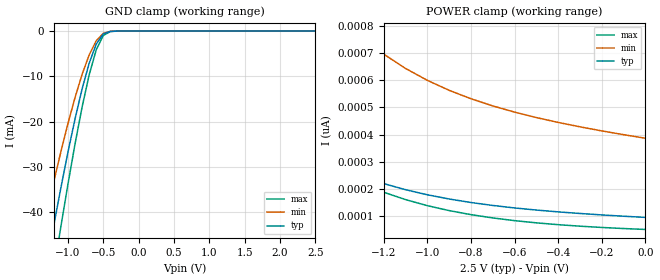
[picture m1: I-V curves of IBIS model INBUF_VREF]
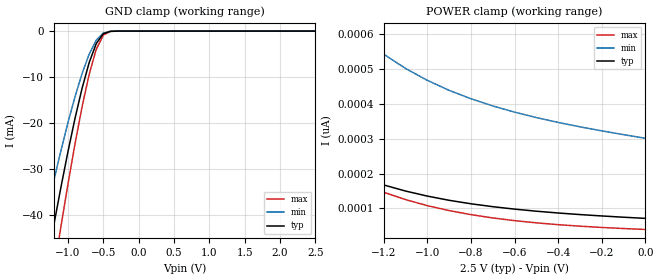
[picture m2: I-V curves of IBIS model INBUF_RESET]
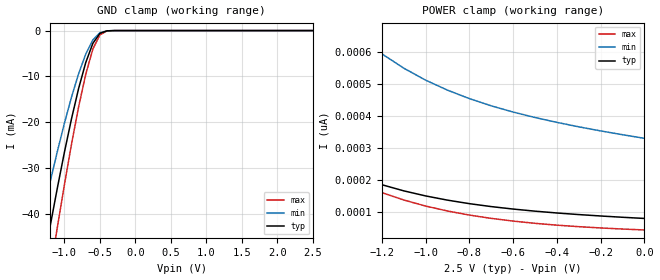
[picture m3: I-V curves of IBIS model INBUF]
| IBIS file sstvn859_mlf_2700.ibs created by s2ibis2 version 1.2
| North Carolina State University Electronics Research Laboratory  1995
[IBIS ver]   2.1
[File name]   sstvn859_mlf_2700.ibs
[File Rev]   1.0
[Date]   Thursday, November 6, 2003
[Source]   IDT
[Notes]   1. Temp typ=25C, min=0C, max=70C
   2. IDT's 2.0v C11.5 process
   3. Ramp rate based on 50 ohm load
READ THESE TERMS AND CONDITIONS CAREFULLY BEFORE USING THIS IBIS MODEL.  BY
USING THIS IBIS MODEL, YOU ARE ACCEPTING AND AGREEING TO THESE TERMS AND
CONDITIONS OF USE.
Integrated Device Technology, Inc. ("IDT") hereby grants the user of this
IBIS model ("User") a non-exclusive, nontransferable license to use this
IBIS model under the following terms: The User is granted this license only
to use the IBIS model for demonstration purposes only and is not granted
rights to sell, copy (except as needed to run the IBIS model), rent, lease
or sub-license (except for demonstration) the IBIS model in whole or in
part, or in modified form to anyone. The User may modify the IBIS model to
suit its specific applications, but  rights to derivative works and such
modifications shall belong to IDT.
THIS IBIS MODEL IS PROVIDED ON AN AS IS" BASIS AND IDT  MAKES ABSOLUTELY NO
WARRANTY WITH RESPECT TO THE INFORMATION CONTAINED HEREIN.  IDT DISCLAIMS
AND USER WAIVES ALL WARRANTIES, EXPRESS AND IMPLIED, INCLUDING WARRANTIES OF
MERCHANTABILITY AND FITNESS FOR A PARTICULAR PURPOSE.  THE ENTIRE RISK AS TO
QUALITY AND PERFORMANCE IS WITH THE USER  ACCORDINGLY, IN NO EVENT SHALL IDT
BE LIABLE FOR ANY DIRECT OR INDIRECT DAMAGES, WHETHER IN CONTRACT OR TORT,
INCLUDING ANY LOST PROFITS OR OTHER INCIDENTAL, CONSEQUENTIAL, EXEMPLARY, OR
PUNITIVE DAMAGES ARISING OUT OF THE USE OR APPLICATION OF THE  IBIS MODEL,
WHETHER OR NOT IDT HAD NOTICE OF SUCH DAMAGES.
IDT reserves the right to make changes without notice to any product herein
to improve reliability, function, or design. IDT does not convey any license
under patent rights or any other intellectual property rights, including
those of third parties. IDT is not obligated to provide maintenance or
support for the licensed IBIS model.
This model is for the 13-Bit to 26-Bit Registered Buffer With SSTL I/O
configuration
[Copyright]
Copyright 2002, Integrated Device Technology, Inc. All rights reserved.
|   Component IDT74SSTVN16859
[Component]   IDT74SSTVN16859
[Manufacturer]   Integrated Device Technology Inc.
[Package]
|Following package parameters are for 56 lead MLF package
| variable   typ   min   max
R_pkg   0.11300   87.30000m   0.15140
L_pkg   2.59000nH   1.99000nH   3.46400nH
C_pkg   0.19900pF   0.15600pF   0.25600pF
[Pin]  signal_name   model_name   R_pin   L_pin   C_pin
1   Q7A   OUTBUF
2   Q6A   OUTBUF
3   Q5A   OUTBUF
4   Q4A   OUTBUF
5   Q3A   OUTBUF
6   Q2A   OUTBUF
7   Q1A   OUTBUF
8   Q13B   OUTBUF
9   VDDQ   POWER
10   Q12B   OUTBUF
11   Q11B   OUTBUF
12   Q10B   OUTBUF
13   Q9B   OUTBUF
14   Q8B   OUTBUF
15   Q7B   OUTBUF
16   Q6B   OUTBUF
17   VDDQ   POWER
18   Q5B   OUTBUF
19   Q4B   OUTBUF
20   Q3B   OUTBUF
21   Q2B   OUTBUF
22   Q1B   OUTBUF
23   VDDQ   POWER
24   D1   INBUF
25   D2   INBUF
26   VDD   POWER
27   VDDQ   POWER
28   D3   INBUF
29   D4   INBUF
30   D5   INBUF
31   D6   INBUF
32   VREF   INBUF_VREF
33   VDD   POWER
34   VDDQ   POWER
35   CLK   INBUF_CLK
36   _CLK_   INBUF_CLK
37   GND   GND
38   _RESET_   INBUF_RESET
39   D7   INBUF
40   D8   INBUF
41   D9   INBUF
42   D10   INBUF
43   D11   INBUF
44   VDDQ   POWER
45   VDD   POWER
46   D12   INBUF
47   D13   INBUF
48   GND   INBUF
49   VDDQ   POWER
50   Q13A   OUTBUF
51   Q12A   OUTBUF
52   Q11A   OUTBUF
53   Q10A   OUTBUF
54   Q9A   OUTBUF
55   VDDQ   POWER
56   Q8A   OUTBUF
| in   in   dummy_model
[Diff Pin]  inv_pin  vdiff   tdelay_typ  tdelay_min  tdelay_max
35   36   0.36000V  NA | CLK/CLKB pins
[Pin Mapping]  pulldown_ref   pullup_ref   gnd_clamp_ref  power_clamp_ref
1   GND   VDDQ
2   GND   VDDQ
3   GND   VDDQ
4   GND   VDDQ
5   GND   VDDQ
6   GND   VDDQ
7   GND   VDDQ
8   GND   VDDQ
9   NC   VDDQ
10   GND   VDDQ
11   GND   VDDQ
12   GND   VDDQ
13   GND   VDDQ
14   GND   VDDQ
15   GND   VDDQ
16   GND   VDDQ
17   NC   VDDQ
18   GND   VDDQ
19   GND   VDDQ
20   GND   VDDQ
21   GND   VDDQ
22   GND   VDDQ
23   NC   VDDQ
24   NC   NC   GND   VDDQ
25   NC   NC   GND   VDDQ
26   NC   VDD
27   NC   VDDQ
28   NC   NC   GND   VDDQ
29   NC   NC   GND   VDDQ
30   NC   NC   GND   VDDQ
31   NC   NC   GND   VDDQ
32   NC   NC   GND   VDDQ
33   NC   VDD
34   NC   VDDQ
35   NC   NC   GND   VDDQ
36   NC   NC   GND   VDDQ
37   GND   NC
38   NC   NC   GND   VDDQ
39   NC   NC   GND   VDDQ
40   NC   NC   GND   VDDQ
41   NC   NC   GND   VDDQ
42   NC   NC   GND   VDDQ
43   NC   NC   GND   VDDQ
44   NC   VDDQ
45   NC   VDD
46   NC   NC   GND   VDDQ
47   NC   NC   GND   VDDQ
48   GND   NC
49   NC   VDDQ
50   GND   VDDQ
51   GND   VDDQ
52   GND   VDDQ
53   GND   VDDQ
54   GND   VDDQ
55   NC   VDDQ
56   GND   VDDQ
| Models and submodels in the file (5): INBUF_VREF (Input), INBUF_RESET (Input), INBUF (Input), INBUF_CLK (Input), OUTBUF (Output)
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|   Model INBUF_VREF
[Model]   INBUF_VREF
Model_type   Input
Polarity   Non-Inverting
Vinl =  1.15000V
Vinh =  1.35000V
C_comp   2.50000pF   2.50000pF   2.50000pF
[Temperature Range]   25.00000   70.00000   0.000
[Voltage Range]   2.50000V   2.30000V   2.70000V
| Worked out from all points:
|   GND clamp passes 1 mA (typ) near -0.52 V on its own axis
[GND_clamp]
| voltage   I(typ)   I(min)   I(max)
-2.5V     -159.7mA   -131mA     -184.7mA
-1.4V     -60.05mA   -47.14mA   -72.86mA
-1.3V     -51.32mA   -40.05mA   -62.76mA
-1.2V     -42.8mA    -33.18mA   -52.81mA
-1.1V     -34.56mA   -26.6mA    -43.11mA
-900mV    -19.37mA   -14.66mA   -24.89mA
-800mV    -12.74mA   -9.544mA   -16.75mA
-700mV    -7.091mA   -5.252mA   -9.645mA
-600mV    -2.871mA   -2.118mA   -4.115mA
-500mV    -637.8uA   -495.3uA   -959.3uA
-300mV    -3.063uA   -4.006uA   -3.923uA
2.5V      94.52pA    413.4pA    44.37pA
[POWER_clamp]
| voltage   I(typ)   I(min)   I(max)
-2.5V     1.398nA    3.51nA     1.623nA
-2.2V     889.8pA    2.286nA    1.003nA
-2.1V     764.4pA    1.985nA    850.6pA
-2V       656.9pA    1.728nA    719.6pA
-1.9V     565.1pA    1.509nA    607.8pA
-1.7V     420.8pA    1.168nA    432.1pA
-1.4V     279.1pA    835.6pA    259.6pA
-1.3V     246.4pA    759.4pA    219.9pA
-1.2V     219.2pA    696.1pA    187.1pA
-1V       177.9pA    599.6pA    137.8pA
-700mV    138.6pA    505.4pA    92.57pA
0V        94.52pA    386.3pA    50.09pA
|   Model INBUF_RESET
[Model]   INBUF_RESET
Model_type   Input
Polarity   Non-Inverting
Vinl =  0.70000V
Vinh =  1.70000V
C_comp   2.50000pF   2.50000pF   2.50000pF
[Temperature Range]   25.00000   70.00000   0.000
[Voltage Range]   2.50000V   2.30000V   2.70000V
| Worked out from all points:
|   GND clamp passes 1 mA (typ) near -0.52 V on its own axis
[GND_clamp]
| voltage   I(typ)   I(min)   I(max)
-2.5V     -158.2mA   -129.5mA   -183.4mA
-1.4V     -59.32mA   -46.36mA   -72.17mA
-1.3V     -50.66mA   -39.34mA   -62.13mA
-1.2V     -42.21mA   -32.55mA   -52.25mA
-1.1V     -34.04mA   -26.05mA   -42.6mA
-900mV    -18.98mA   -14.27mA   -24.51mA
-800mV    -12.43mA   -9.231mA   -16.44mA
-700mV    -6.859mA   -5.022mA   -9.408mA
-600mV    -2.718mA   -1.972mA   -3.951mA
-500mV    -567.1uA   -431.8uA   -874.7uA
-300mV    -2.396uA   -3.132uA   -3.069uA
2.5V      70.97pA    322.6pA    34.6pA
[POWER_clamp]
| voltage   I(typ)   I(min)   I(max)
-2.5V     1.086nA    2.739nA    1.267nA
-2.2V     689.4pA    1.783nA    783.1pA
-2.1V     591.6pA    1.549nA    663.8pA
-2V       507.7pA    1.348nA    561.6pA
-1.9V     436.2pA    1.178nA    474.3pA
-1.7V     323.8pA    911.3pA    337.2pA
-1.4V     213.5pA    651.9pA    202.5pA
-1.3V     188.1pA    592.5pA    171.6pA
-1.2V     167pA      543.1pA    146pA
-1V       135pA      467.8pA    107.5pA
-700mV    104.6pA    394.3pA    72.21pA
0V        70.97pA    301.3pA    39.06pA
|   Model INBUF
[Model]   INBUF
Model_type   Input
Polarity   Non-Inverting
Vinl =  0.84000V
Vinh =  1.66000V
C_comp   2.50000pF   2.50000pF   2.50000pF
[Temperature Range]   25.00000   70.00000   0.000
[Voltage Range]   2.50000V   2.30000V   2.70000V
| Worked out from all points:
|   GND clamp passes 1 mA (typ) near -0.52 V on its own axis
[GND_clamp]
| voltage   I(typ)   I(min)   I(max)
-2.5V     -159.1mA   -130.4mA   -184.2mA
-1.4V     -59.73mA   -46.79mA   -72.56mA
-1.3V     -51.03mA   -39.73mA   -62.48mA
-1.2V     -42.53mA   -32.89mA   -52.56mA
-1.1V     -34.32mA   -26.35mA   -42.88mA
-900mV    -19.19mA   -14.47mA   -24.71mA
-800mV    -12.59mA   -9.39mA    -16.6mA
-700mV    -6.975mA   -5.134mA   -9.529mA
-600mV    -2.79mA    -2.039mA   -4.03mA
-500mV    -596.8uA   -457.6uA   -911.7uA
-300mV    -2.619uA   -3.425uA   -3.355uA
2.5V      78.81pA    352.8pA    37.85pA
[POWER_clamp]
| voltage   I(typ)   I(min)   I(max)
-2.5V     1.19nA     2.996nA    1.386nA
-2.2V     756.2pA    1.951nA    856.5pA
-2.1V     649.2pA    1.694nA    726.1pA
-2V       557.4pA    1.475nA    614.3pA
-1.9V     479.1pA    1.288nA    518.8pA
-1.7V     356.2pA    996.8pA    368.8pA
-1.4V     235.3pA    713.1pA    221.5pA
-1.3V     207.5pA    648.1pA    187.7pA
-1.2V     184.4pA    594.1pA    159.7pA
-1V       149.3pA    511.7pA    117.6pA
-700mV    115.9pA    431.3pA    79pA
0V        78.81pA    329.6pA    42.73pA
